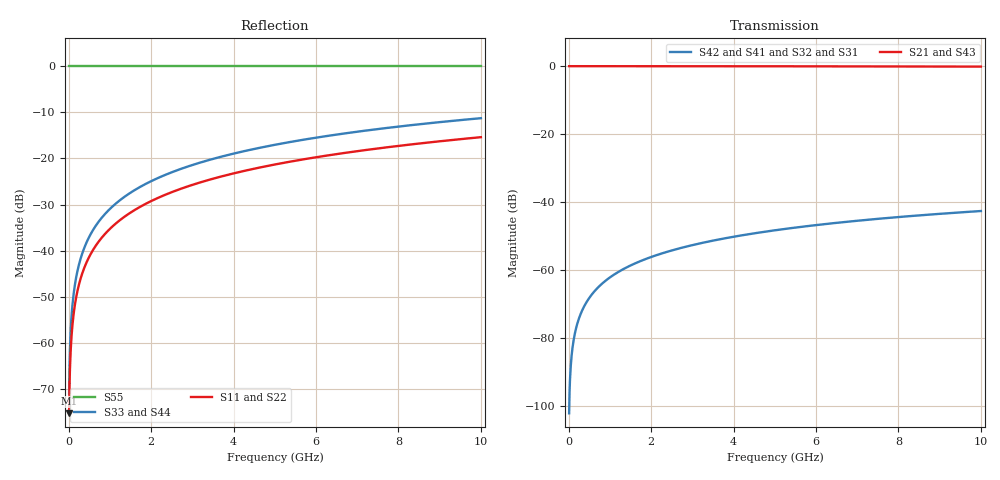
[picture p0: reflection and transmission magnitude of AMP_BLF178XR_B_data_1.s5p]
! Created Mon Oct  5 17:54:15 2009
# ghz S ma R 50
! 5 Port Network Data from SP1.SP block
! freq  magS11  angS11  magS12  angS12  magS13  angS13  magS14  angS14
!  magS15  angS15
!  magS21  angS21  magS22  angS22  magS23  angS23
!  magS24  angS24  magS25  angS25
!  magS31  angS31  magS32  angS32
!  magS33  angS33  magS34  angS34  magS35  angS35
!  magS41  angS41
!  magS42  angS42  magS43  angS43  magS44  angS44  magS45  angS45
!  magS51  angS51  magS52  angS52  magS53  angS53  magS54  angS54
!  magS55  angS55
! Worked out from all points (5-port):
!   1000 points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, 10 MHz to 10 GHz, reference 50 ohm
!   strongest paths, dB at 10 MHz, 2.51 GHz, 5.01 GHz, 7.51 GHz, 10 GHz:
!     S21: 0.0, 0.0, 0.0, -0.1, -0.1
!     S43: 0.0, 0.0, -0.1, -0.2, -0.3
!     S42: -102.2, -54.2, -48.3, -44.9, -42.6
!     S41: -102.2, -54.2, -48.3, -44.9, -42.6
!     S32: -102.2, -54.2, -48.3, -44.9, -42.6
!     S31: -102.2, -54.2, -48.3, -44.9, -42.6
!   lowest |S11| = -75.3 dB at 10 MHz (marker M1), VSWR 1.00, Z = 50 + j0.0172 ohm
!   |S11| at or under -10 dB: start of sweep to end of sweep
